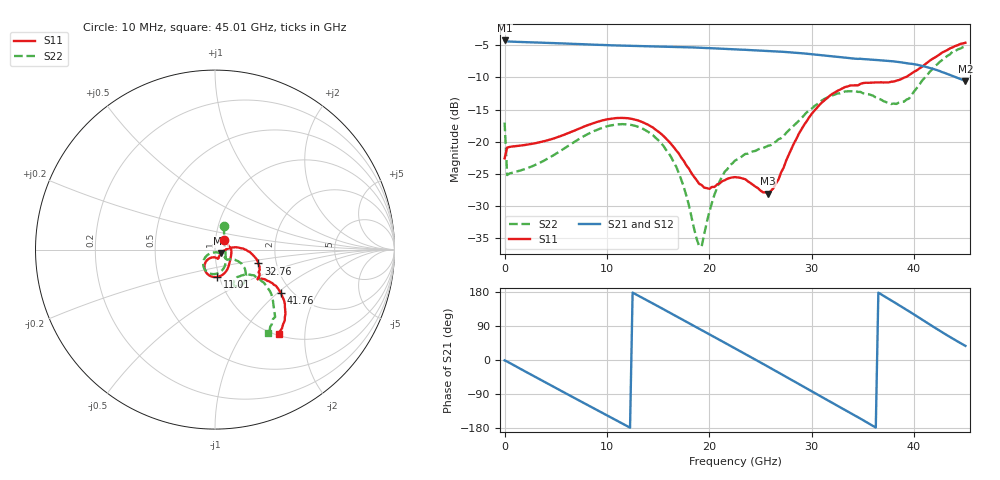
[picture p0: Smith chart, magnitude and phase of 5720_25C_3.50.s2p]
! Device:  ADRF5720
! Description: 0.5dB LSB GaAs MMIC 6-bit Digital Attenuator
! Frequency:  0.000009 -  40 GHz
! Ports:
!	RF1	= Port 1
!	RF2	= Port 2
! Vdd:  3.3 Volt
! Vss:  -3.3 Volt
! Control:  0/3.3 Volt
! State:  3.50 dB attenuation
! Data:  The device was measured using G-S-G Probes on a matrix board.
!  Data was collected using an calibrated 4 port network analyzer.
!  The reference plane for this measurement is at the launchers.
! Note:  Analog Devices supplies this data as a sample of measured data
!  for this product.  Your particular data for this product may vary.
!  Data was taken at 25 degrees C.
!  Analog Devices reserves the right to change this data at anytime.
# GHZ S DB R 45.0
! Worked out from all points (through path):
!   181 points, 10 MHz to 45.01 GHz, reference 45 ohm
!   highest |S21| = -4.26 dB at 10 MHz (marker M1); lowest = -10.6 dB at 45.01 GHz (marker M2)
!   group delay of S21, straight-line fit = 41.8 ps
!   lowest |S11| = -28.1 dB at 25.76 GHz (marker M3), VSWR 1.08, Z = 48 - j2.06 ohm
!   |S11| at or under -10 dB: start of sweep to 39.1 GHz
!   |S22| runs from -36.2 to -5.2 dB; largest |S21 - S12| = 0.0007
!   S11 on the Smith chart (normalised r, x): 10 MHz: 1.10, +0.12; 11.01 GHz: 0.98, -0.30; 32.76 GHz: 1.61, -0.27; 41.76 GHz: 1.75, -1.05; 45.01 GHz: 1.03, -1.47
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0.01  -22.57 45.0  -4.26 -1.0  -4.27 -1.0  -17.02 69.8
0.26  -20.91 1.1  -4.41 -4.1  -4.41 -4.1  -25.18 3.2
2.01  -20.50 -17.1  -4.52 -30.1  -4.52 -30.1  -24.23 -17.6
4.26  -19.75 -35.0  -4.64 -62.9  -4.64 -62.9  -22.58 -36.4
7.76  -17.65 -59.0  -4.85 -113.7  -4.85 -113.7  -19.13 -62.2
11.01  -16.31 -85.9  -5.04 -160.5  -5.04 -160.5  -17.30 -91.3
13.26  -16.83 -105.7  -5.13 167.0  -5.13 167.0  -17.81 -113.5
15.26  -18.73 -120.3  -5.20 137.8  -5.20 137.8  -20.17 -132.1
17.26  -22.46 -127.2  -5.29 108.5  -5.29 108.5  -25.89 -144.4
19.01  -26.54 -112.3  -5.39 82.6  -5.39 82.6  -36.22 -91.2
19.26  -26.74 -107.8  -5.40 78.9  -5.40 78.9  -36.23 -74.2
21.01  -26.49 -79.8  -5.52 53.0  -5.52 53.0  -26.16 -34.9
22.76  -25.54 -71.7  -5.66 26.9  -5.66 27.0  -22.70 -38.7
25.76  -28.08 -32.9  -5.90 -17.9  -5.90 -17.9  -20.62 -36.3
28.26  -20.27 6.8  -6.15 -55.9  -6.15 -55.9  -17.49 -26.9
30.26  -15.17 -0.6  -6.43 -86.5  -6.44 -86.5  -14.47 -31.3
32.76  -11.91 -17.7  -6.84 -124.6  -6.84 -124.5  -12.47 -46.3
35.26  -10.83 -30.9  -7.17 -162.6  -7.17 -162.5  -12.57 -60.0
37.76  -10.68 -34.0  -7.48 157.6  -7.48 157.6  -14.14 -54.7
39.51  -9.64 -30.7  -7.85 128.4  -7.85 128.4  -13.29 -39.6
41.76  -7.16 -33.5  -8.63 89.8  -8.63 89.8  -8.76 -36.1
45.01  -4.62 -52.9  -10.55 37.3  -10.54 37.4  -5.19 -57.2
